TYPE Warning :
STRUCT
	//PRESSURE_Alarm:BOOL;
	PRESSURE:BOOL;
	
	//MFC1_Alarm:BOOL;
	MFC1:BOOL;
	
	//MFC2_Alarm:BOOL;
	MFC2:BOOL;
	
	//MFC3_Alarm:BOOL;
	MFC3:BOOL;
	
	//MFC4_Alarm:BOOL;
	MFC4:BOOL;
	
	//MFC5_Alarm:BOOL;
	MFC5:BOOL;
	
	//MFC6_Alarm:BOOL;
	MFC6:BOOL;
	
	//MFC7_Alarm:BOOL;
	MFC7:BOOL;
	
	//MFC8_Alarm:BOOL;
	MFC8:BOOL;
	
	//MFC9_Alarm:BOOL;
	MFC9:BOOL;
	
	//WALL_TEMP_Alarm:BOOL;
	WALL_TEMP:BOOL;
	
	//LID_TEMP_Alarm:BOOL;
	LID_TEMP:BOOL;
	
	//STAGE_TEMP_Warning:BOOL;	
	STAGE_TEMP1:BOOL;
	STAGE_TEMP2:BOOL;
	STAGE_TEMP3:BOOL;
	STAGE_TEMP4:BOOL;
	
	
	
	OpenCloseSlitValveTimeout:BOOL;
	Gas1FlowPressureOutOfRange:BOOL;
	Gas2FlowPressureOutOfRange:BOOL;
	Gas3FlowPressureOutOfRange:BOOL;
	Gas4FlowPressureOutOfRange:BOOL;
	Gas5FlowPressureOutOfRange:BOOL;
	Gas6FlowPressureOutOfRange:BOOL;
	Gas7FlowPressureOutOfRange:BOOL;
	Gas8FlowPressureOutOfRange:BOOL;
	Gas9FlowPressureOutOfRange:BOOL;	
	
	
	//PROCESS TOLERANCE
	TOLERANCE_PRESSURE:BOOL;
	TOLERANCE_MFC1:BOOL;
	TOLERANCE_MFC2:BOOL;
	TOLERANCE_MFC3:BOOL;
	TOLERANCE_MFC4:BOOL;
	TOLERANCE_MFC5:BOOL;
	TOLERANCE_MFC6:BOOL;
	TOLERANCE_MFC7:BOOL;
	TOLERANCE_MFC8:BOOL;
	TOLERANCE_MFC9:BOOL;
	TOLERANCE_WALL_TEMP:BOOL;
	TOLERANCE_LID_TEMP:BOOL;
	TOLERANCE_STAGE_TEMP1,
	TOLERANCE_STAGE_TEMP2,
	TOLERANCE_STAGE_TEMP3,
	TOLERANCE_STAGE_TEMP4: BOOL;	
	

END_STRUCT
END_TYPE
